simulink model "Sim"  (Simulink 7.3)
settings: Solver=ode45  StartTime=0.0  StopTime=150  RelTol=1e-3
undefined symbols (not defined in the file or in its folder): Av, Bv, Cv, Dv, Kmix, Kpr, Kq

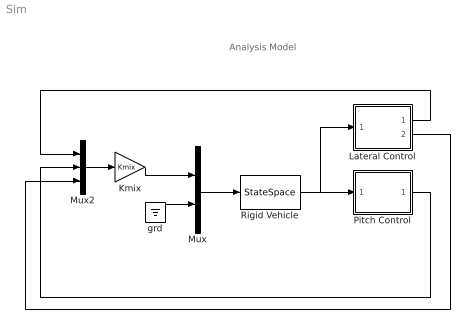
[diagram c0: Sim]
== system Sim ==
  note: Analysis Model
  Kmix : Gain  Gain=Kmix  Multiplication=Matrix(K*u)  ParameterDataType=fixdt(1, 16)  ParameterScaling=2^0  OutDataType=fixdt(1, 16)  OutScaling=2^0
  Lateral Control : Subsystem
  Mux : Mux  Inputs=[4,1]
  Mux2 : Mux  Inputs=3
  Pitch Control : Subsystem
  Rigid Vehicle : StateSpace  A=Av  B=Bv  C=Cv  D=Dv
  grd : Ground
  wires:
  Mux/1 -> Rigid Vehicle/1
  Kmix/1 -> Mux/1
  grd/1 -> Mux/2
  Rigid Vehicle/1 -> Pitch Control/1(xp), Lateral Control/1(xl)
  Mux2/1 -> Kmix/1
  Pitch Control/1(DQ) -> Mux2/2
  Lateral Control/1(DP) -> Mux2/1
  Lateral Control/2(DR) -> Mux2/3

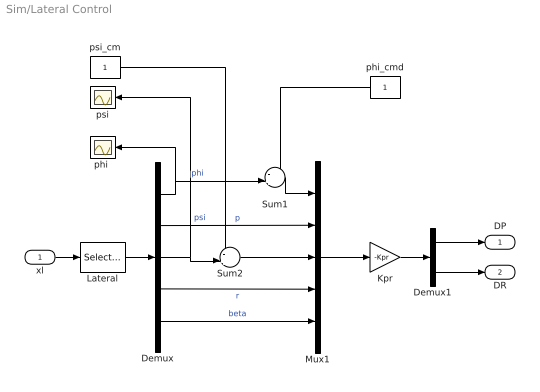
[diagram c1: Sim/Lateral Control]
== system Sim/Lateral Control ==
  xl : Inport
  Demux : Demux  Outputs=5
  Demux1 : Demux  Outputs=2
  Kpr : Gain  Gain=-Kpr  Multiplication=Matrix(K*u)  ParameterDataType=fixdt(1, 16)  ParameterScaling=2^0  OutDataType=fixdt(1, 16)  OutScaling=2^0
  Lateral : Selector  InputPortWidth=14  IndexOptions=Index vector (dialog)  Indices=[1,2, 5,6, 8]  OutputSizes=1
  Mux1 : Mux  Inputs=5
  Sum1 : Sum  Inputs=-+|  OutDataType=sfix(16)  OutScaling=2^0
  Sum2 : Sum  Inputs=-+|  OutDataType=sfix(16)  OutScaling=2^0
  "phi " : Scope
  phi_cmd : Constant  OutDataType=fixdt(1, 16)  OutScaling=2^0
  psi : Scope
  psi_cm : Constant  OutDataType=fixdt(1, 16)  OutScaling=2^0
  DP : Outport
  DR : Outport  Port=2
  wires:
  Demux/2 -> Mux1/2  "p"
  Lateral/1 -> Demux/1
  Mux1/1 -> Kpr/1
  xl/1 -> Lateral/1
  Demux/4 -> Mux1/4  "r"
  psi_cm/1 -> Sum2/1
  Demux/5 -> Mux1/5  "beta"
  Demux/3 -> Sum2/2, psi/1  "psi"
  Sum2/1 -> Mux1/3
  Kpr/1 -> Demux1/1
  Demux1/1 -> DP/1
  Demux1/2 -> DR/1
  Sum1/1 -> Mux1/1
  Demux/1 -> Sum1/2, "phi "/1  "phi"
  phi_cmd/1 -> Sum1/1

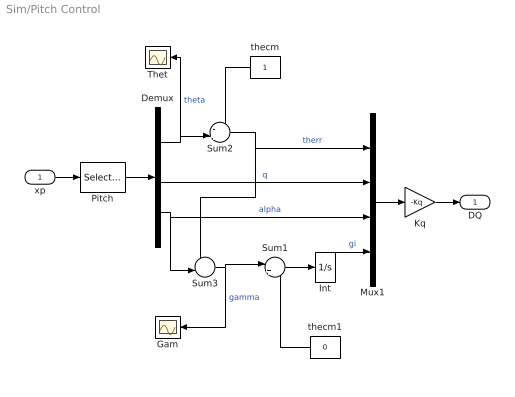
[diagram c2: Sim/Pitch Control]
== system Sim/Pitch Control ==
  xp : Inport
  Demux : Demux  Outputs=3
  Gam : Scope
  Int : Integrator
  Kq : Gain  Gain=-Kq  Multiplication=Matrix(K*u)  ParameterDataType=fixdt(1, 16)  ParameterScaling=2^0  OutDataType=fixdt(1, 16)  OutScaling=2^0
  Mux1 : Mux
  Pitch : Selector  InputPortWidth=14  IndexOptions=Index vector (dialog)  Indices=[3, 4, 7]  OutputSizes=1
  Sum1 : Sum  Inputs=|+-  OutDataType=sfix(16)  OutScaling=2^0
  Sum2 : Sum  Inputs=-+|  OutDataType=sfix(16)  OutScaling=2^0
  Sum3 : Sum  Inputs=+-|  OutDataType=sfix(16)  OutScaling=2^0
  Thet : Scope
  thecm : Constant  OutDataType=fixdt(1, 16)  OutScaling=2^0
  thecm1 : Constant  Value=0  OutDataType=fixdt(1, 16)  OutScaling=2^0
  DQ : Outport
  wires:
  Demux/2 -> Mux1/2  "q"
  Demux/3 -> Mux1/3, Sum3/2  "alpha"
  Pitch/1 -> Demux/1
  Mux1/1 -> Kq/1
  Demux/1 -> Sum2/2, Thet/1  "theta"
  Sum2/1 -> Mux1/1, Sum3/1  "therr"
  thecm/1 -> Sum2/1
  xp/1 -> Pitch/1
  Kq/1 -> DQ/1
  Int/1 -> Mux1/4  "gi"
  thecm1/1 -> Sum1/2
  Sum1/1 -> Int/1
  Sum3/1 -> Sum1/1, Gam/1  "gamma"
